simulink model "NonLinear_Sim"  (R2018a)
settings: Solver=ode4  StartTime=0.0  StopTime=32000  FixedStep=Ts  MaxStep=0.5  RelTol=1e-3  EnableMultiTasking=on
InitFcn:
  | run
StopFcn:
  | pl
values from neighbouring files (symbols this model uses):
  Cw2b = [ 0,          0,          0    [run.m]
  d2r = pi/180    (= 0.0174532925199)    [run.m]    (also in runf.m; orbitic.m; Quan.m)
  ini = [wb0; atto; Hco]    [run.m]
  Kq1 = I22*ww^2 - 3*wo2*(I11-I33)    [run.m]
  Kq2 = 2*I22*zet*ww    [run.m]
  Kqi = 0.0005    [run.m]
  Kr1 = (0.1*I11*I33*zet^2/Hy0) - sqrt( ((0.01^zet^4*I11^2*I33^2)/Hy0^2)+(4*I11*I33*zet^2) )    [run.m]
  Kr2 = 0.05*Kr1    [run.m]
  Kr3 = 0.04*zet*(Kr2-Hy0) * sqrt(abs(Hy0/(I11*I33)))    [run.m]
  nt = 7    [run.m]    (also in runf.m)
  Tmax = 0.05    [run.m]
  Ts = 0.001    [run.m]    (also in runf.m = 0.0005)
  wo = Worb    [run.m]
undefined symbols (not defined in the file or in its folder): DiscIntNeverNeededParam, Mode_Switch, NonLin_Vehi_Dynamics, Phase_Plane, RW_Steering
libraries: simulink x4

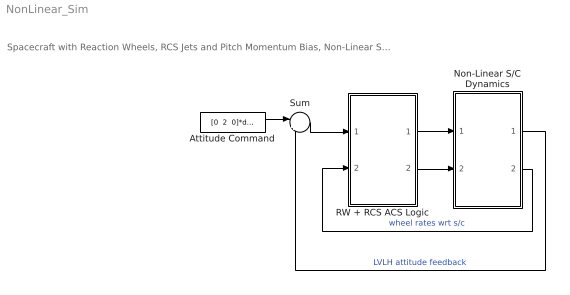
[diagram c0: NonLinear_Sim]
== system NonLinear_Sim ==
  note: Spacecraft with Reaction Wheels, RCS Jets and Pitch Momentum Bias, Non-Linear Simulation
  Attitude Command : Constant  Value="[0  2  0]*d2r"
  Non-Linear S/C Dynamics : Subsystem
  RW + RCS ACS Logic : Subsystem
  Sum : Sum  Inputs=|+-
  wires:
  Non-Linear S/C Dynamics/2(wr) -> RW + RCS ACS Logic/2(wr(i))  "wheel rates wrt s/c"
  Attitude Command/1 -> Sum/1
  Non-Linear S/C Dynamics/1(att-lv) -> Sum/2  "LVLH attitude feedback"
  Sum/1 -> RW + RCS ACS Logic/1(atter)
  RW + RCS ACS Logic/2(Trwi) -> Non-Linear S/C Dynamics/2(Twi)
  RW + RCS ACS Logic/1(Frcs) -> Non-Linear S/C Dynamics/1(Frcs)

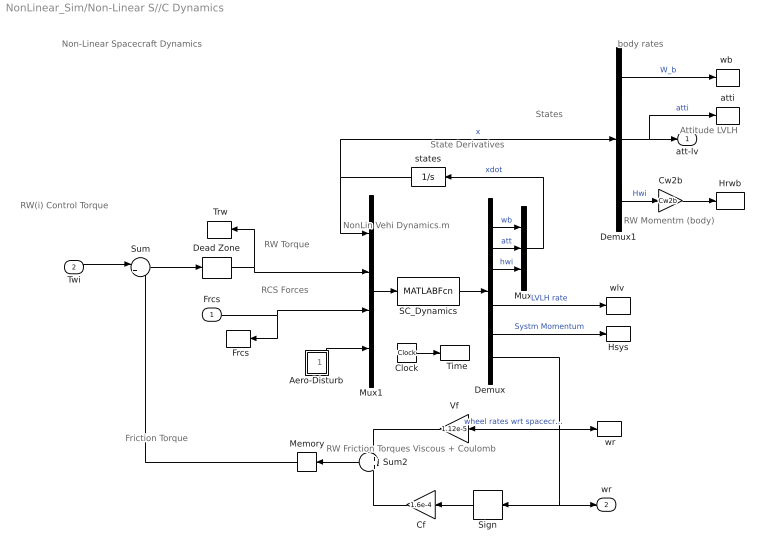
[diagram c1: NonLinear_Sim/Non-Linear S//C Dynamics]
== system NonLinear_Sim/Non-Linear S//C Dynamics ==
  note: Non-Linear Spacecraft Dynamics
  note: State Derivatives
  note: body rates
  note: RCS Forces
  note: Friction Torque
  note: States
  note: RW Friction Torques Viscous + Coulomb
  note: Attitude LVLH
  note: RW Torque
  note: RW(i) Control Torque
  note: RW Momentm (body)
  note: NonLin Vehi Dynamics.m
  Frcs : Inport  PortDimensions=nt
  Twi : Inport  Port=2
  "  Frcs" : ToWorkspace  VariableName=Frcs  SampleTime=-1
  "  Time" : ToWorkspace  VariableName=time  SampleTime=-1
  " Trw" : ToWorkspace  VariableName=Trw  SampleTime=-1
  " wr" : ToWorkspace  VariableName=wr  SampleTime=-1
  Aero-Disturb : Subsystem
  Cf : Gain  Gain=1.6e-4
  Clock : Clock
  Cw2b : Gain  Gain=Cw2b  Multiplication=Matrix(K*u)
  Dead Zone : DeadZone  LowerValue=-[1, 1, 1]*Tmax/1000  UpperValue=[1 1 1]*Tmax/1000
  Demux : Demux  Outputs="[3,3,3,  3,3,3]"
  Demux1 : Demux  Outputs=[3,3,3]
  Hrwb : ToWorkspace  VariableName=Hrwb  SampleTime=-1
  Hsys : ToWorkspace  VariableName=Hsys  SampleTime=-1
  Memory : Memory
  Mux : Mux  Inputs=[3,3,3]
  Mux1 : Mux  Inputs=[9,3, nt, 3]
  SC_Dynamics : MATLABFcn  MATLABFcn=NonLin_Vehi_Dynamics( u(1:9), u(10:12), u(13:12+nt), u(13+nt:15+nt) )  OutputDimensions=9+9
  Sign : Signum
  Sum : Sum  Inputs=|+-
  Sum2 : Sum  Inputs=+|+
  Vf : Gain  Gain=1.12e-5
  atti : ToWorkspace  VariableName=atti  SampleTime=-1
  states : Integrator  InitialCondition=ini
  "wb " : ToWorkspace  VariableName=wb  SampleTime=-1
  "wlv " : ToWorkspace  VariableName=wlv  SampleTime=-1
  att-lv : Outport
  wr : Outport  Port=2
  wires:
  Demux/6 -> wr/1, Sign/1, Vf/1, " wr"/1  "wheel rates wrt spacecrft"
  Demux1/3 -> Cw2b/1  "Hwi"
  Demux/5 -> Hsys/1  "Systm Momentum"
  Demux/4 -> "wlv "/1  "LVLH rate"
  Demux1/2 -> att-lv/1, atti/1  "atti"
  Mux1/1 -> SC_Dynamics/1
  SC_Dynamics/1 -> Demux/1
  Clock/1 -> "  Time"/1
  Frcs/1 -> Mux1/3, "  Frcs"/1
  Demux/3 -> Mux/3  "hwi"
  Demux1/1 -> "wb "/1  "W_b"
  states/1 -> Demux1/1, Mux1/1  "x"
  Demux/2 -> Mux/2  "att"
  Demux/1 -> Mux/1  "wb"
  Vf/1 -> Sum2/1
  Sign/1 -> Cf/1
  Cf/1 -> Sum2/2
  Twi/1 -> Sum/1
  Sum/1 -> Dead Zone/1
  Memory/1 -> Sum/2
  Dead Zone/1 -> Mux1/2, " Trw"/1
  Sum2/1 -> Memory/1
  Cw2b/1 -> Hrwb/1
  Mux/1 -> states/1  "xdot"
  Aero-Disturb/1(Td) -> Mux1/4

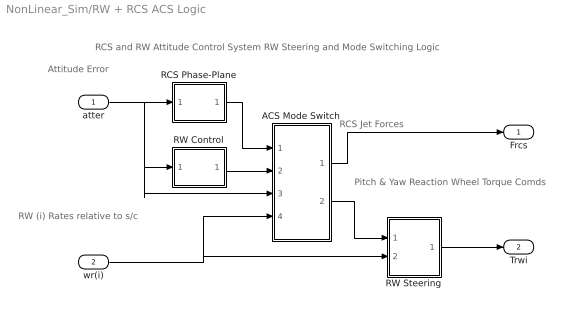
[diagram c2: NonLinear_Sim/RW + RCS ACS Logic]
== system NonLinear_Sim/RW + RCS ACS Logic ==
  note: RCS and RW Attitude Control System RW Steering and Mode Switching Logic
  note: RCS Jet Forces
  note: RW (i) Rates relative to s/c
  note: Attitude Error
  note: Pitch & Yaw Reaction Wheel Torque Comds
  atter : Inport
  wr(i) : Inport  Port=2
  ACS Mode Switch : Subsystem
  RCS Phase-Plane : Subsystem
  RW Control : Subsystem
  RW Steering : Subsystem
  Frcs : Outport
  Trwi : Outport  Port=2
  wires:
  atter/1 -> RCS Phase-Plane/1(atter), ACS Mode Switch/3(atter), RW Control/1(atti)
  RCS Phase-Plane/1(f(nt)) -> ACS Mode Switch/1(Frcs)
  wr(i)/1 -> RW Steering/2(wr(1)), ACS Mode Switch/4(wr(i))
  ACS Mode Switch/1(" Frcs") -> Frcs/1
  RW Steering/1(Twi) -> Trwi/1
  RW Control/1(Tc) -> ACS Mode Switch/2(Trw)
  ACS Mode Switch/2(" Trw") -> RW Steering/1(Trwc)

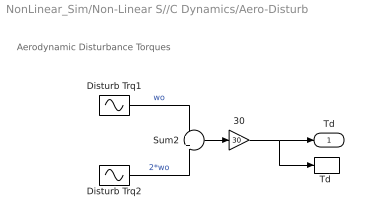
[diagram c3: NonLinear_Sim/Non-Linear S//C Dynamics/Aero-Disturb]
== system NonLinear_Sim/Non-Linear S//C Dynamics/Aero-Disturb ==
  note: Aerodynamic Disturbance Torques
  30 : Gain  Gain=30
  Disturb Trq1 : Sin  Amplitude="[0.0,  1.2,  0.4]*0.0001"  Bias="[0.0,  0.6,  0.2]*0.0001"  Frequency=[wo, wo, wo]  SampleTime=0
  Disturb Trq2 : Sin  Amplitude=[0, 1.2, 1]*0.0001  Bias="[0  0.2  0.1]*0.0001"  Frequency=[wo, wo, wo]*2  SampleTime=0
  Sum2 : Sum  Inputs=+|+
  "Td " : ToWorkspace  VariableName=Td  SampleTime=-1
  Td : Outport
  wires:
  30/1 -> "Td "/1, Td/1
  Disturb Trq2/1 -> Sum2/2  "2*wo"
  Sum2/1 -> 30/1
  Disturb Trq1/1 -> Sum2/1  "wo"

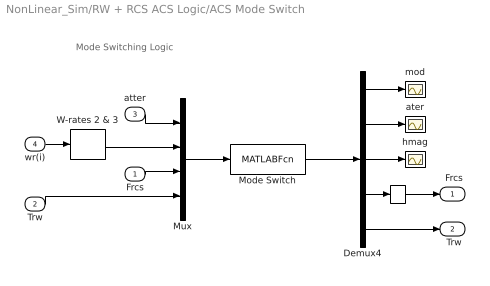
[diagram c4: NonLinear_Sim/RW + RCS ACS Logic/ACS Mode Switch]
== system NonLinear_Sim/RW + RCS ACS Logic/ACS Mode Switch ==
  note: Mode Switching Logic
  Frcs : Inport
  Trw : Inport  Port=2
  atter : Inport  Port=3
  wr(i) : Inport  Port=4
  "   " : Memory
  Demux4 : Demux  Outputs="[1 1 1 nt  2]"
  Mode Switch : MATLABFcn  MATLABFcn=Mode_Switch( u(1:3), u(4:5), u(6:5+nt), u(6+nt:7+nt) )  OutputDimensions=3+nt+2
  Mux : Mux  Inputs="[3  2  nt 2]"
  W-rates 2 & 3 : Selector  InputPortWidth=3  IndexOptions=Index vector (dialog)  Indices="[2  3]"  OutputSizes=1
  ater : Scope
  hmag : Scope
  mod : Scope
  " Frcs" : Outport
  " Trw" : Outport  Port=2
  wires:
  atter/1 -> Mux/1
  Mux/1 -> Mode Switch/1
  wr(i)/1 -> W-rates 2 & 3/1
  Frcs/1 -> Mux/3
  Trw/1 -> Mux/4
  Mode Switch/1 -> Demux4/1
  Demux4/4 -> "   "/1
  Demux4/5 -> " Trw"/1
  Demux4/1 -> mod/1
  Demux4/2 -> ater/1
  Demux4/3 -> hmag/1
  "   "/1 -> " Frcs"/1
  W-rates 2 & 3/1 -> Mux/2

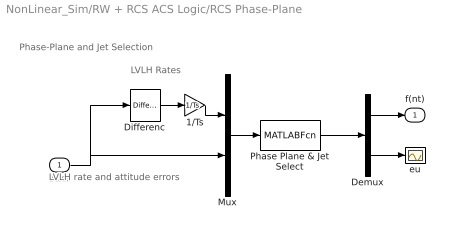
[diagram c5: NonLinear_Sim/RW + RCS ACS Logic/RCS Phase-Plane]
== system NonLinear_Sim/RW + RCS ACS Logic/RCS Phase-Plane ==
  note: Phase-Plane and Jet Selection
  note: LVLH rate and attitude errors
  note: LVLH Rates
  atter : Inport
  1/Ts : Gain  Gain=1/Ts
  Demux : Demux  Outputs=[nt, 3]
  Differenc : simulink/Discrete/Difference  ICPrevInput=0.0  InputProcessing=Inherited  OutMin=[]  OutMax=[]  OutDataType=sfix(16)  OutScaling=2^-10  DoSatur=off
  Mux : Mux  Inputs="[3  3]"
  Phase Plane & Jet Select : MATLABFcn  MATLABFcn=Phase_Plane( u(1:3), u(4:6) )  OutputDimensions=nt + 3
  eu : Scope
  f(nt) : Outport
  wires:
  atter/1 -> Mux/2, Differenc/1
  1/Ts/1 -> Mux/1
  Demux/2 -> eu/1
  Demux/1 -> f(nt)/1
  Phase Plane & Jet Select/1 -> Demux/1
  Mux/1 -> Phase Plane & Jet Select/1
  Differenc/1 -> 1/Ts/1

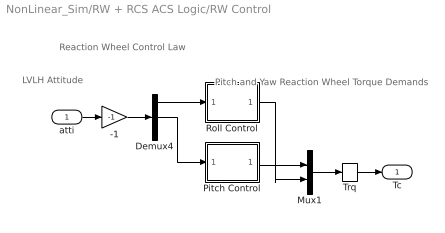
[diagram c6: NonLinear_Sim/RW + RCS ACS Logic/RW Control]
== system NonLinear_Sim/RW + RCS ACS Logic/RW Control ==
  note: Pitch and Yaw Reaction Wheel Torque Demands
  note: LVLH Attitude
  note: Reaction Wheel Control Law
  atti : Inport
  -1 : Gain  Gain=-1
  Demux4 : Demux  Outputs=3
  Mux1 : Mux  Inputs=2
  Pitch Control : Subsystem
  Roll Control : Subsystem
  Trq : Memory
  Tc : Outport
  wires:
  Demux4/1 -> Roll Control/1(phi)
  Pitch Control/1(Tcy) -> Mux1/1
  Demux4/2 -> Pitch Control/1(the)
  atti/1 -> -1/1
  Mux1/1 -> Trq/1
  -1/1 -> Demux4/1
  Roll Control/1(Tcz) -> Mux1/2
  Trq/1 -> Tc/1

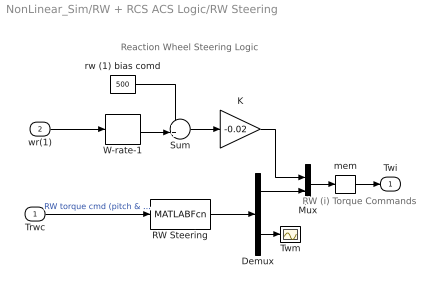
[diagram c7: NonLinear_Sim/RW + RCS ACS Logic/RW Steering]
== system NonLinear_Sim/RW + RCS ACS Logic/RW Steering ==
  note: RW (i) Torque Commands
  note: Reaction Wheel Steering Logic
  Trwc : Inport
  wr(1) : Inport  Port=2
  Demux : Demux  Outputs=[2, 1]
  K : Gain  Gain=-0.02
  Mux : Mux  Inputs=[1,2]
  RW Steering : MATLABFcn  MATLABFcn=RW_Steering( u(1:2) )  OutputDimensions=3
  Sum : Sum  Inputs=++|
  Twm : Scope
  W-rate-1 : Selector  InputPortWidth=3  IndexOptions=Index vector (dialog)  Indices=[1]  OutputSizes=1
  mem : Memory
  rw (1) bias comd : Constant  Value=500
  Twi : Outport
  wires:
  Demux/2 -> Twm/1
  Demux/1 -> Mux/2
  RW Steering/1 -> Demux/1
  Trwc/1 -> RW Steering/1  "RW torque cmd (pitch & yaw)"
  Mux/1 -> mem/1
  wr(1)/1 -> W-rate-1/1
  Sum/1 -> K/1
  rw (1) bias comd/1 -> Sum/1
  W-rate-1/1 -> Sum/2
  K/1 -> Mux/1
  mem/1 -> Twi/1

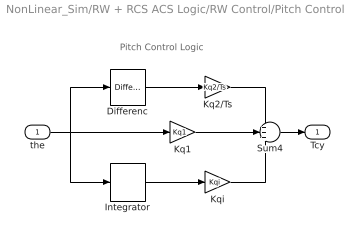
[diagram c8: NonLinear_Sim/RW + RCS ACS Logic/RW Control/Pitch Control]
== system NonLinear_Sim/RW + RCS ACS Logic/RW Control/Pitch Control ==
  note: Pitch Control Logic
  the : Inport
  Differenc : simulink/Discrete/Difference  ICPrevInput=0.0  InputProcessing=Inherited  OutMin=[]  OutMax=[]  OutDataType=sfix(16)  OutScaling=2^-10  DoSatur=off
  Integrator : DiscreteIntegrator  SampleTime=Ts  ICPrevOutput=DiscIntNeverNeededParam  ICPrevScaledInput=DiscIntNeverNeededParam
  Kq1 : Gain  Gain=Kq1
  Kq2/Ts : Gain  Gain=Kq2/Ts
  Kqi : Gain  Gain=Kqi
  Sum4 : Sum  Inputs=+++
  Tcy : Outport
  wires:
  Kq1/1 -> Sum4/2
  Sum4/1 -> Tcy/1
  Kq2/Ts/1 -> Sum4/1
  the/1 -> Kq1/1, Integrator/1, Differenc/1
  Kqi/1 -> Sum4/3
  Integrator/1 -> Kqi/1
  Differenc/1 -> Kq2/Ts/1

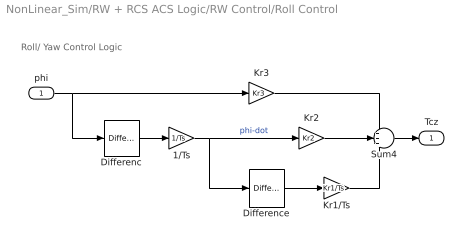
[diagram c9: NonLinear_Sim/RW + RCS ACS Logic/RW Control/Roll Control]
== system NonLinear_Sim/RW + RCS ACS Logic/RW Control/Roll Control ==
  note: Roll/ Yaw Control Logic
  phi : Inport
  1/Ts : Gain  Gain=1/Ts
  Differenc : simulink/Discrete/Difference  ICPrevInput=0.0  InputProcessing=Inherited  OutMin=[]  OutMax=[]  OutDataType=sfix(16)  OutScaling=2^-10  DoSatur=off
  Difference : simulink/Discrete/Difference  ICPrevInput=0.0  InputProcessing=Inherited  OutMin=[]  OutMax=[]  OutDataType=sfix(16)  OutScaling=2^-10  DoSatur=off
  Kr1/Ts : Gain  Gain=Kr1/Ts
  Kr2 : Gain  Gain=Kr2
  Kr3 : Gain  Gain=Kr3
  Sum4 : Sum  Inputs=+++
  Tcz : Outport
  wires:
  Kr3/1 -> Sum4/1
  Kr2/1 -> Sum4/2
  Kr1/Ts/1 -> Sum4/3
  phi/1 -> Kr3/1, Differenc/1
  Sum4/1 -> Tcz/1
  Difference/1 -> Kr1/Ts/1
  Differenc/1 -> 1/Ts/1
  1/Ts/1 -> Kr2/1, Difference/1  "phi-dot"
